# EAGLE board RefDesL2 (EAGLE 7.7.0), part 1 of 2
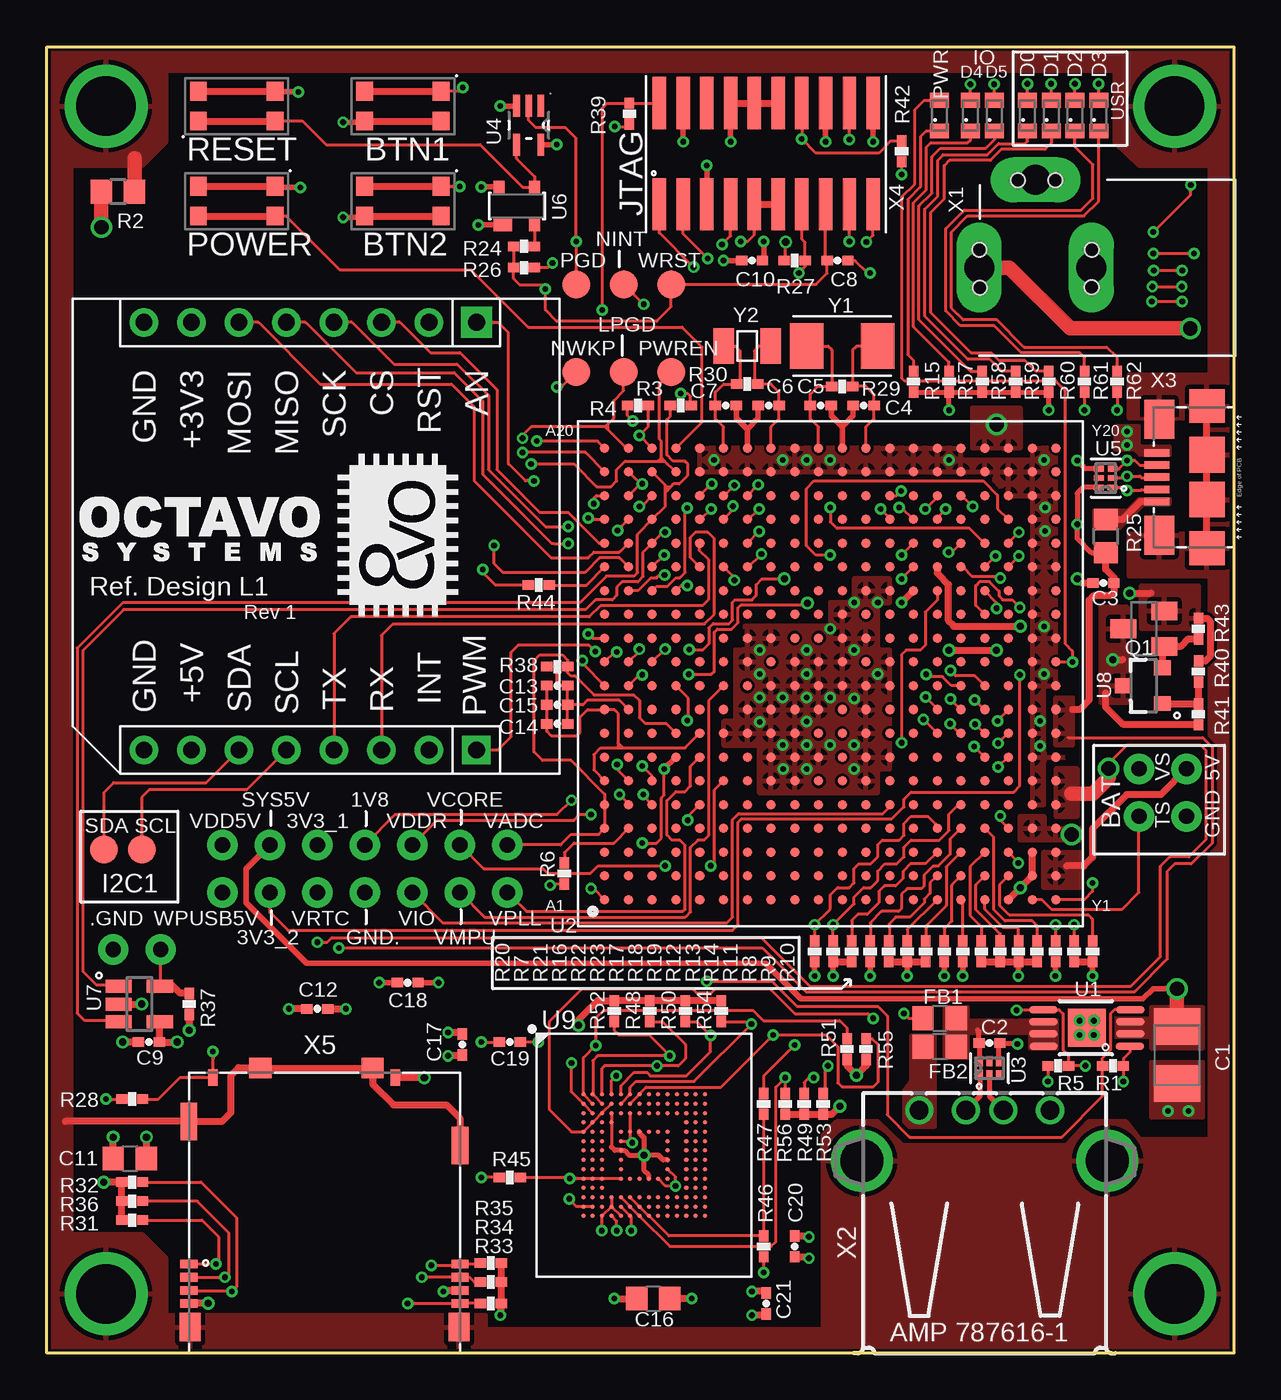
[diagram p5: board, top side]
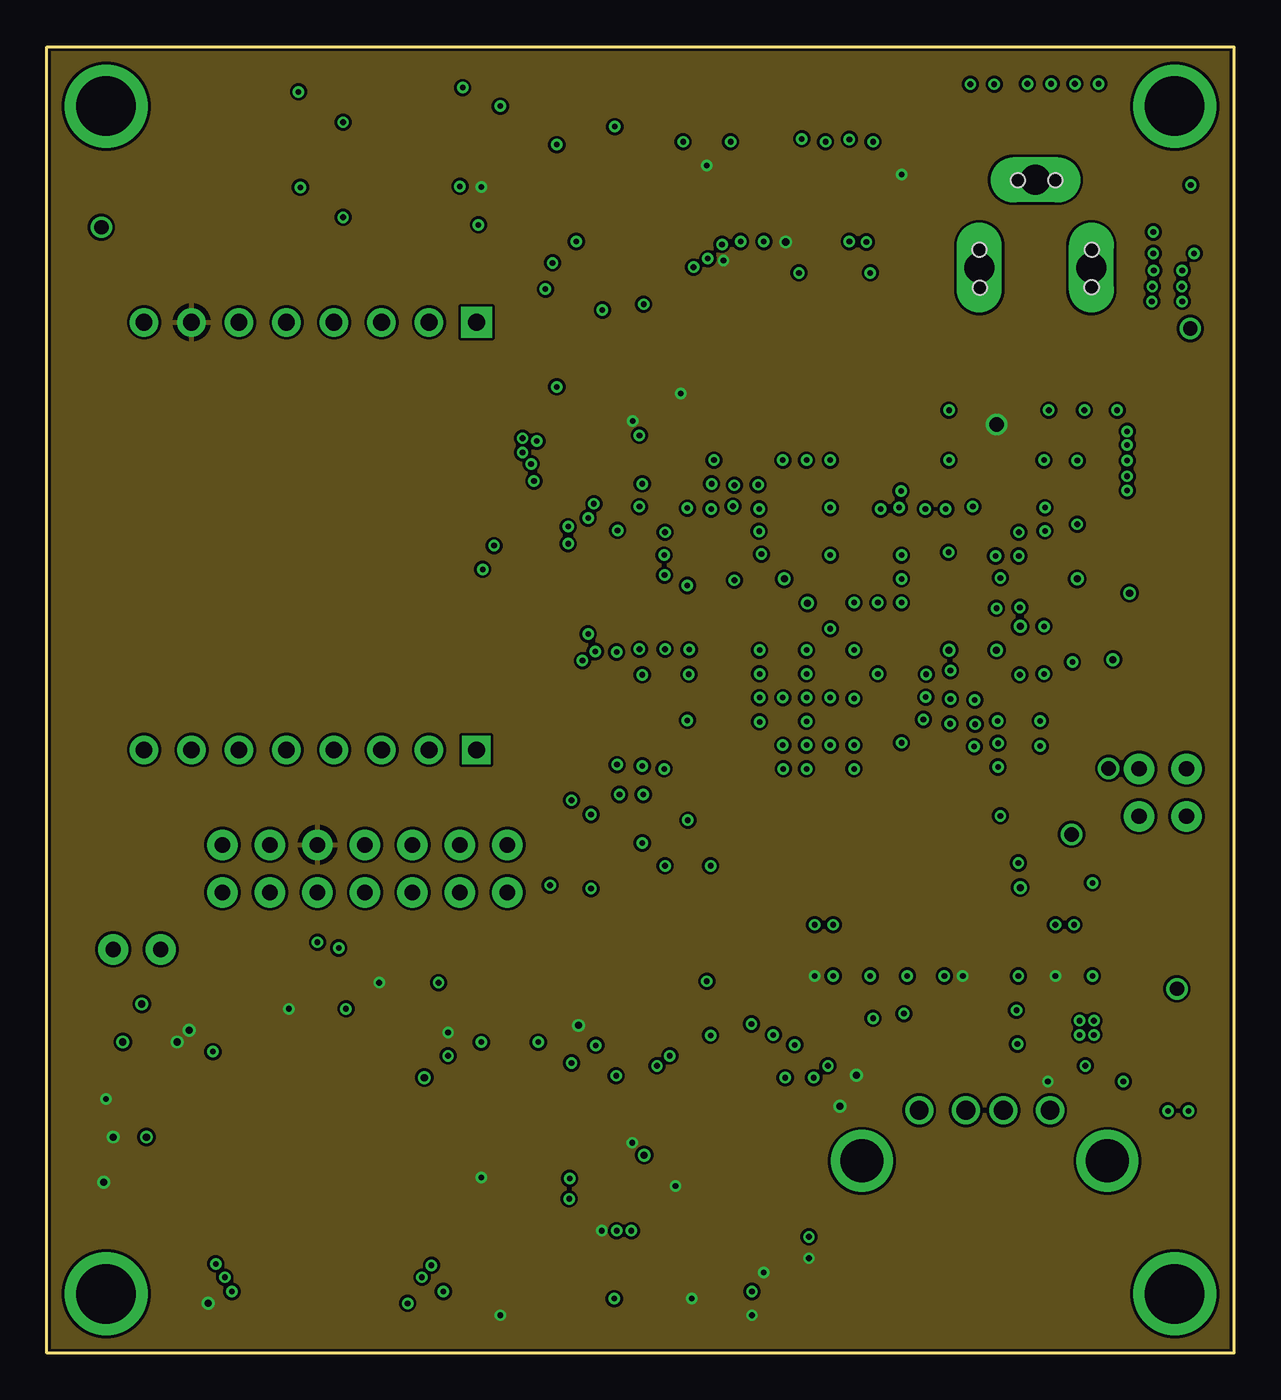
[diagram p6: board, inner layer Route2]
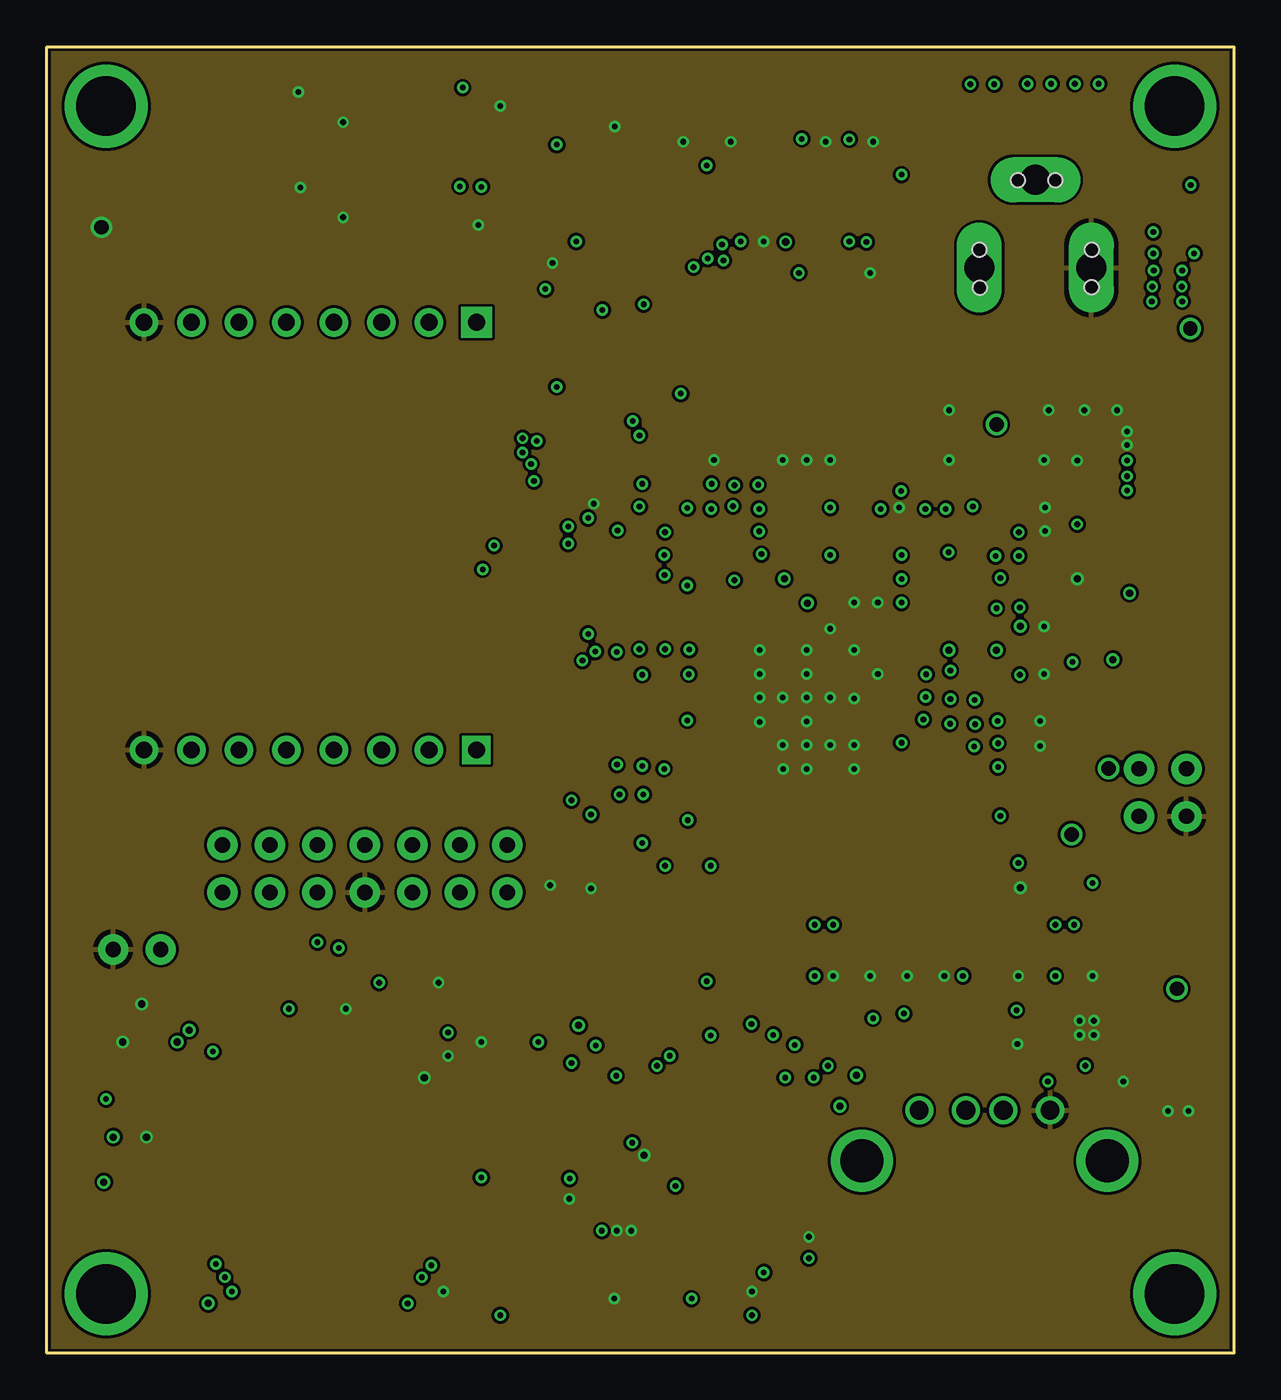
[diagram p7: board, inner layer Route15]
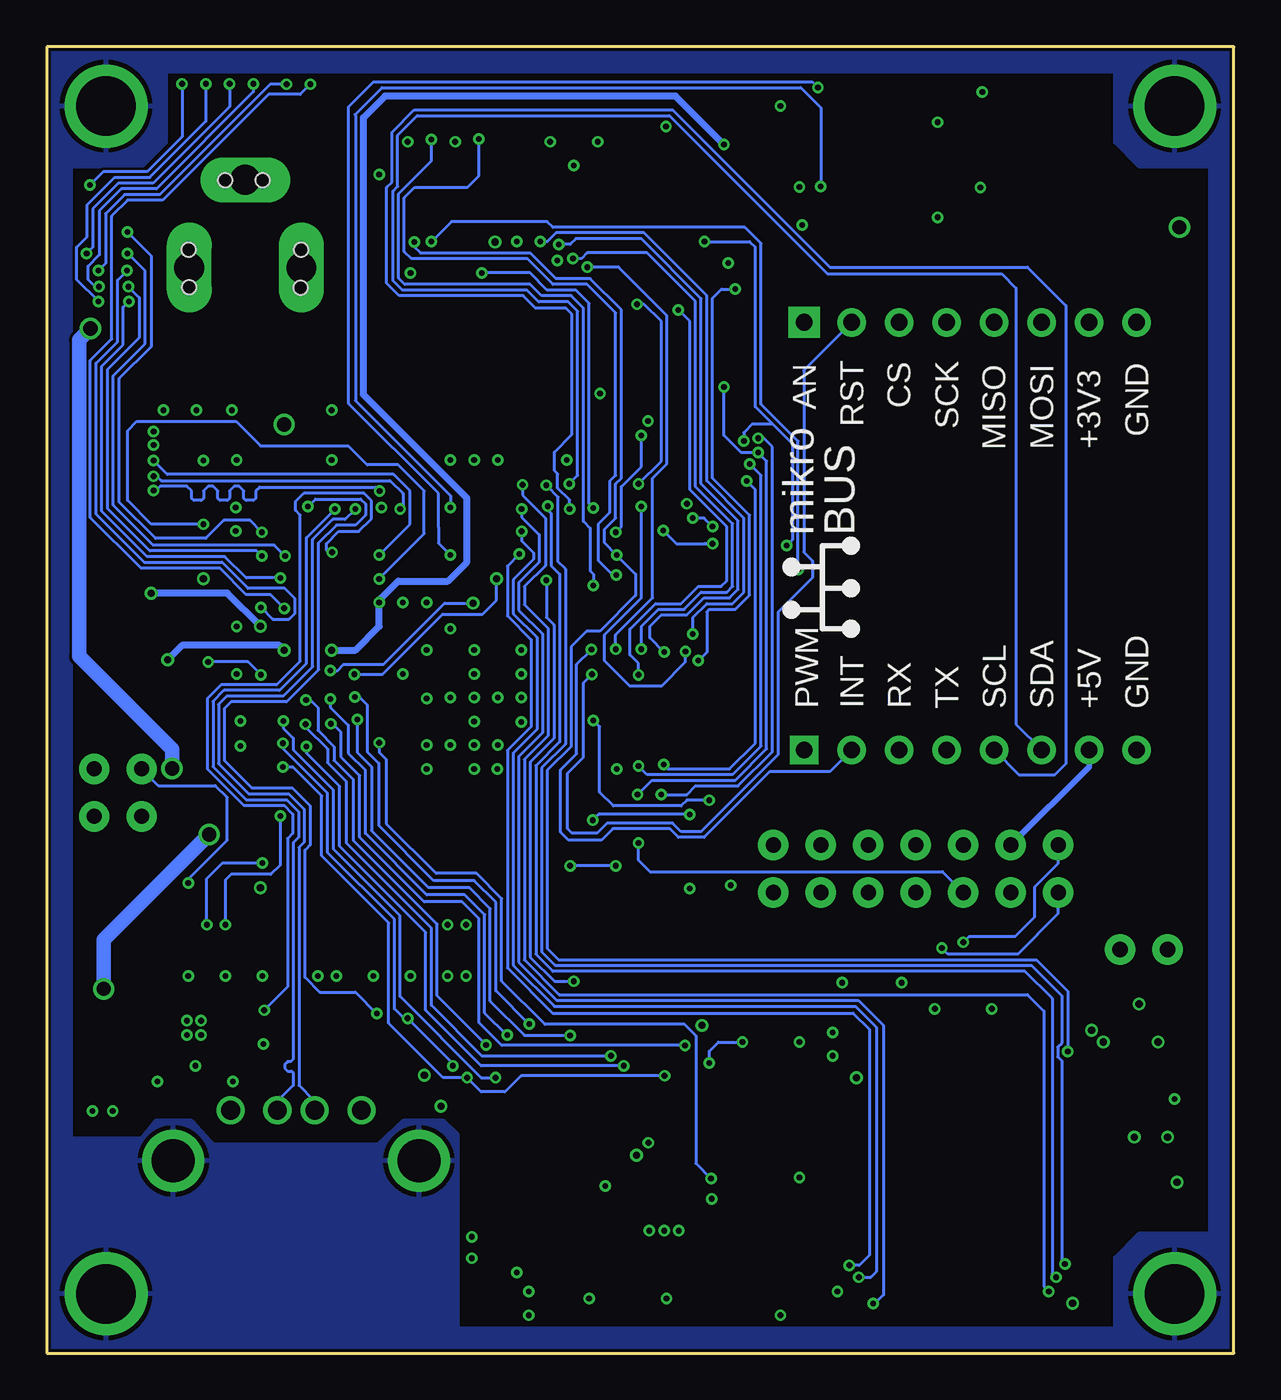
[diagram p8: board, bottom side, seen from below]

Size 63.5 x 69.85 mm. Coordinates in mm from the lower left corner, seen from the top.
Outline: 0,69.85 63.5,69.85 63.5,0 0,0 0,69.85
Copper layers (1+2*15+16): Top 0.07mm / dielectric 0.23mm / Route2 0.035mm / dielectric 0.93mm / Route15 0.035mm / dielectric 0.23mm / Bottom 0.07mm
Design rules "default *": minimum track width 6mil, minimum drill 12mil, track to track 6mil, track to pad 6mil, pad to pad 6mil, via to via 6mil, smd to smd 0mil, copper to edge 6mil, drill to drill 6mil, minimum pad ring 6mil, minimum via ring 6mil, stop-mask expansion 2mil, vias tented up to drill 25mil, thermal gap 10mil
Net classes: 0 default: width 0.127 mm, drill 0.254 mm

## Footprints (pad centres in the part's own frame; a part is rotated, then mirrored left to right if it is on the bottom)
TESTPAD/W_HOLE_1X1 = drill 0.813 pad 1.626: P$1 0,0
SW4SMD_63X161LS = smd 0.9 x 1: 1 2.05,0.8; 2 2.05,-0.8; 3 -2.05,0.8; 4 -2.05,-0.8
B/3528-21R = smd 1.95 x 2.5: + 1.525,0; - -1.525,0
C0402 = smd 0.61 x 0.508: 1 -0.559,0; 2 0.559,0
C0805 = smd 1.143 x 1.27: 1 -0.889,0; 2 0.889,0
EIA-STD = smd 0.787 x 1.016: 1 -0.826,0; 2 0.826,0
TP15R = smd 1.5 x 1.5: TP 0,0
MOUNTING_HOLE = drill 3.175 pad 4.445: P$1 0,0
SOT23-BEC = smd 1 x 1.4: B -0.95,-1.1; C 0,1.1; E 0.95,-1.1
R0402 = smd 0.61 x 0.508: 1 -0.559,0; 2 0.559,0
R0805 = smd 1.143 x 1.27: 1 -0.889,0; 2 0.889,0
S-PDSO-G08 = smd 1.524 x 0.406: 1 -2.311,0.975; 2 -2.324,0.325; 3 -2.324,-0.325; 4 -2.324,-0.975; 5 2.324,-0.975; 6 2.324,-0.325; 7 2.324,0.325; 8 2.311,0.975 | smd 2.032 x 2.032: TH 0,0
OSD335X-BGA-400 = smd 0.5 x 0.5: A1 -12.065,-12.065; A2 -12.065,-10.795; A3 -12.065,-9.525; A4 -12.065,-8.255; A5 -12.065,-6.985; A6 -12.065,-5.715; A7 -12.065,-4.445; A8 -12.065,-3.175; A9 -12.065,-1.905; A10 -12.065,-0.635; A11 -12.065,0.635; A12 -12.065,1.905; A13 -12.065,3.175; A14 -12.065,4.445; A15 -12.065,5.715; A16 -12.065,6.985; A17 -12.065,8.255; A18 -12.065,9.525; A19 -12.065,10.795; A20 -12.065,12.065; B1 -10.795,-12.065; B2 -10.795,-10.795; B3 -10.795,-9.525; B4 -10.795,-8.255; B5 -10.795,-6.985; B6 -10.795,-5.715; B7 -10.795,-4.445; B8 -10.795,-3.175; B9 -10.795,-1.905; B10 -10.795,-0.635; B11 -10.795,0.635; B12 -10.795,1.905; B13 -10.795,3.175; B14 -10.795,4.445; B15 -10.795,5.715; B16 -10.795,6.985; B17 -10.795,8.255; B18 -10.795,9.525; B19 -10.795,10.795; B20 -10.795,12.065; C1 -9.525,-12.065; C2 -9.525,-10.795; C3 -9.525,-9.525; C4 -9.525,-8.255; C5 -9.525,-6.985; C6 -9.525,-5.715; C7 -9.525,-4.445; C8 -9.525,-3.175; C9 -9.525,-1.905; C10 -9.525,-0.635; C11 -9.525,0.635; C12 -9.525,1.905; C13 -9.525,3.175; C14 -9.525,4.445; C15 -9.525,5.715; C16 -9.525,6.985; C17 -9.525,8.255; C18 -9.525,9.525; C19 -9.525,10.795; C20 -9.525,12.065; D1 -8.255,-12.065; D2 -8.255,-10.795; D3 -8.255,-9.525; D4 -8.255,-8.255; D5 -8.255,-6.985; D6 -8.255,-5.715; D7 -8.255,-4.445; D8 -8.255,-3.175; D9 -8.255,-1.905; D10 -8.255,-0.635; D11 -8.255,0.635; D12 -8.255,1.905; D13 -8.255,3.175; D14 -8.255,4.445; D15 -8.255,5.715; D16 -8.255,6.985; D17 -8.255,8.255; D18 -8.255,9.525; D19 -8.255,10.795; D20 -8.255,12.065; E1 -6.985,-12.065; E2 -6.985,-10.795; E3 -6.985,-9.525; E4 -6.985,-8.255; E5 -6.985,-6.985; E6 -6.985,-5.715; E7 -6.985,-4.445; E8 -6.985,-3.175; E9 -6.985,-1.905; E10 -6.985,-0.635; E11 -6.985,0.635; E12 -6.985,1.905; E13 -6.985,3.175; E14 -6.985,4.445; E15 -6.985,5.715; E16 -6.985,6.985; E17 -6.985,8.255; E18 -6.985,9.525; E19 -6.985,10.795; E20 -6.985,12.065; F1 -5.715,-12.065; F2 -5.715,-10.795; F3 -5.715,-9.525; F4 -5.715,-8.255; F5 -5.715,-6.985; F6 -5.715,-5.715; F7 -5.715,-4.445; F8 -5.715,-3.175; F9 -5.715,-1.905; F10 -5.715,-0.635; F11 -5.715,0.635; F12 -5.715,1.905; F13 -5.715,3.175; F14 -5.715,4.445; F15 -5.715,5.715; F16 -5.715,6.985; F17 -5.715,8.255; F18 -5.715,9.525; F19 -5.715,10.795; F20 -5.715,12.065; G1 -4.445,-12.065; G2 -4.445,-10.795; G3 -4.445,-9.525; G4 -4.445,-8.255; G5 -4.445,-6.985; G6 -4.445,-5.715; G7 -4.445,-4.445; G8 -4.445,-3.175; G9 -4.445,-1.905; G10 -4.445,-0.635; G11 -4.445,0.635; G12 -4.445,1.905; G13 -4.445,3.175; G14 -4.445,4.445; G15 -4.445,5.715; G16 -4.445,6.985; G17 -4.445,8.255; G18 -4.445,9.525; G19 -4.445,10.795; G20 -4.445,12.065; H1 -3.175,-12.065; H2 -3.175,-10.795; H3 -3.175,-9.525; H4 -3.175,-8.255; H5 -3.175,-6.985; H6 -3.175,-5.715; H7 -3.175,-4.445; H8 -3.175,-3.175; H9 -3.175,-1.905; H10 -3.175,-0.635; H11 -3.175,0.635; H12 -3.175,1.905; H13 -3.175,3.175; H14 -3.175,4.445; H15 -3.175,5.715; H16 -3.175,6.985; H17 -3.175,8.255; H18 -3.175,9.525; H19 -3.175,10.795; H20 -3.175,12.065; J1 -1.905,-12.065; J2 -1.905,-10.795; J3 -1.905,-9.525; J4 -1.905,-8.255; J5 -1.905,-6.985; J6 -1.905,-5.715; J7 -1.905,-4.445; J8 -1.905,-3.175; J9 -1.905,-1.905; J10 -1.905,-0.635; J11 -1.905,0.635; J12 -1.905,1.905; J13 -1.905,3.175; J14 -1.905,4.445; J15 -1.905,5.715; J16 -1.905,6.985; J17 -1.905,8.255; J18 -1.905,9.525; J19 -1.905,10.795; J20 -1.905,12.065; K1 -0.635,-12.065; K2 -0.635,-10.795; K3 -0.635,-9.525; K4 -0.635,-8.255; K5 -0.635,-6.985; K6 -0.635,-5.715; K7 -0.635,-4.445; K8 -0.635,-3.175; K9 -0.635,-1.905; K10 -0.635,-0.635; K11 -0.635,0.635; K12 -0.635,1.905; K13 -0.635,3.175; K14 -0.635,4.445; K15 -0.635,5.715; K16 -0.635,6.985; K17 -0.635,8.255; K18 -0.635,9.525; K19 -0.635,10.795; K20 -0.635,12.065; L1 0.635,-12.065; L2 0.635,-10.795; L3 0.635,-9.525; L4 0.635,-8.255; L5 0.635,-6.985; L6 0.635,-5.715; L7 0.635,-4.445; L8 0.635,-3.175; L9 0.635,-1.905; L10 0.635,-0.635; L11 0.635,0.635; L12 0.635,1.905; L13 0.635,3.175; L14 0.635,4.445; L15 0.635,5.715; L16 0.635,6.985; L17 0.635,8.255; L18 0.635,9.525; L19 0.635,10.795; L20 0.635,12.065; M1 1.905,-12.065; M2 1.905,-10.795; M3 1.905,-9.525; M4 1.905,-8.255; M5 1.905,-6.985; M6 1.905,-5.715; M7 1.905,-4.445; M8 1.905,-3.175; M9 1.905,-1.905; M10 1.905,-0.635; M11 1.905,0.635; M12 1.905,1.905; M13 1.905,3.175; M14 1.905,4.445; M15 1.905,5.715; M16 1.905,6.985; M17 1.905,8.255; M18 1.905,9.525; M19 1.905,10.795; M20 1.905,12.065; N1 3.175,-12.065; N2 3.175,-10.795; N3 3.175,-9.525; N4 3.175,-8.255; N5 3.175,-6.985; N6 3.175,-5.715; N7 3.175,-4.445; N8 3.175,-3.175; N9 3.175,-1.905; N10 3.175,-0.635; N11 3.175,0.635; N12 3.175,1.905; N13 3.175,3.175; N14 3.175,4.445; N15 3.175,5.715; N16 3.175,6.985; N17 3.175,8.255; N18 3.175,9.525; N19 3.175,10.795; N20 3.175,12.065; P1 4.445,-12.065; P2 4.445,-10.795; P3 4.445,-9.525; P4 4.445,-8.255; P5 4.445,-6.985; P6 4.445,-5.715; P7 4.445,-4.445; P8 4.445,-3.175; P9 4.445,-1.905; P10 4.445,-0.635; P11 4.445,0.635; P12 4.445,1.905; P13 4.445,3.175; P14 4.445,4.445; P15 4.445,5.715; P16 4.445,6.985; P17 4.445,8.255; P18 4.445,9.525; P19 4.445,10.795; P20 4.445,12.065; R1 5.715,-12.065; R2 5.715,-10.795; R3 5.715,-9.525; R4 5.715,-8.255; R5 5.715,-6.985; R6 5.715,-5.715; R7 5.715,-4.445; R8 5.715,-3.175; R9 5.715,-1.905; R10 5.715,-0.635; R11 5.715,0.635; R12 5.715,1.905; R13 5.715,3.175; R14 5.715,4.445; R15 5.715,5.715; R16 5.715,6.985; R17 5.715,8.255; R18 5.715,9.525; R19 5.715,10.795; R20 5.715,12.065; T1 6.985,-12.065; T2 6.985,-10.795; T3 6.985,-9.525; T4 6.985,-8.255; T5 6.985,-6.985; T6 6.985,-5.715; T7 6.985,-4.445; T8 6.985,-3.175; T9 6.985,-1.905; T10 6.985,-0.635; T11 6.985,0.635; T12 6.985,1.905; T13 6.985,3.175; T14 6.985,4.445; T15 6.985,5.715; T16 6.985,6.985; T17 6.985,8.255; T18 6.985,9.525; T19 6.985,10.795; T20 6.985,12.065; U1 8.255,-12.065; U2 8.255,-10.795; U3 8.255,-9.525; U4 8.255,-8.255; U5 8.255,-6.985; U6 8.255,-5.715; U7 8.255,-4.445; U8 8.255,-3.175; U9 8.255,-1.905; U10 8.255,-0.635; U11 8.255,0.635; U12 8.255,1.905; U13 8.255,3.175; U14 8.255,4.445; U15 8.255,5.715; U16 8.255,6.985; U17 8.255,8.255; U18 8.255,9.525; U19 8.255,10.795; U20 8.255,12.065; V1 9.525,-12.065; V2 9.525,-10.795; V3 9.525,-9.525; V4 9.525,-8.255; V5 9.525,-6.985; V6 9.525,-5.715; V7 9.525,-4.445; V8 9.525,-3.175; V9 9.525,-1.905; V10 9.525,-0.635; V11 9.525,0.635; V12 9.525,1.905; V13 9.525,3.175; V14 9.525,4.445; V15 9.525,5.715; V16 9.525,6.985; V17 9.525,8.255; V18 9.525,9.525; V19 9.525,10.795; V20 9.525,12.065; W1 10.795,-12.065; W2 10.795,-10.795; W3 10.795,-9.525; W4 10.795,-8.255; W5 10.795,-6.985; W6 10.795,-5.715; W7 10.795,-4.445; W8 10.795,-3.175; W9 10.795,-1.905; W10 10.795,-0.635; W11 10.795,0.635; W12 10.795,1.905; W13 10.795,3.175; W14 10.795,4.445; W15 10.795,5.715; W16 10.795,6.985; W17 10.795,8.255; W18 10.795,9.525; W19 10.795,10.795; W20 10.795,12.065; Y1 12.065,-12.065; Y2 12.065,-10.795; Y3 12.065,-9.525; Y4 12.065,-8.255; Y5 12.065,-6.985; Y6 12.065,-5.715; Y7 12.065,-4.445; Y8 12.065,-3.175; Y9 12.065,-1.905; Y10 12.065,-0.635; Y11 12.065,0.635; Y12 12.065,1.905; Y13 12.065,3.175; Y14 12.065,4.445; Y15 12.065,5.715; Y16 12.065,6.985; Y17 12.065,8.255; Y18 12.065,9.525; Y19 12.065,10.795; Y20 12.065,12.065
DRY6 = smd 0.55 x 0.3: 1 -0.355,0.5 | smd 0.52 x 0.3: 2 -0.37,0; 3 -0.37,-0.5; 4 0.37,-0.5; 5 0.37,0; 6 0.37,0.5
DCK5 = smd 1.168 x 0.356: 1 -1.041,0.65; 2 -1.041,0; 3 -1.041,-0.65; 4 1.041,-0.65; 5 1.041,0.65
SOT143-R = smd 1 x 0.7: 1 -0.75,-1 | smd 0.6 x 0.7: 2 0.95,-1; 3 0.95,1; 4 -0.95,1
SOT23-5 = smd 0.7 x 1.4: 1 0.95,1.1; 2 0,1.1; 3 -0.95,1.1; 4 -0.95,-1.1; 5 0.95,-1.1
SOT23-3 = smd 0.8 x 0.9: 1 -0.95,-1; 2 0.95,-1; 3 0,1.1
MICRON_EMMC_153 = smd 0.245 x 0.245: A1 -3.25,3.25; A2 -2.75,3.25; A3 -2.25,3.25; A4 -1.75,3.25; A5 -1.25,3.25; A6 -0.75,3.25; A7 -0.25,3.25; A8 0.25,3.25; A9 0.75,3.25; A10 1.25,3.25; A11 1.75,3.25; A12 2.25,3.25; A13 2.75,3.25; A14 3.25,3.25; B1 -3.25,2.75; B2 -2.75,2.75; B3 -2.25,2.75; B4 -1.75,2.75; B5 -1.25,2.75; B6 -0.75,2.75; B7 -0.25,2.75; B8 0.25,2.75; B9 0.75,2.75; B10 1.25,2.75; B11 1.75,2.75; B12 2.25,2.75; B13 2.75,2.75; B14 3.25,2.75; C1 -3.25,2.25; C2 -2.75,2.25; C3 -2.25,2.25; C4 -1.75,2.25; C5 -1.25,2.25; C6 -0.75,2.25; C7 -0.25,2.25; C8 0.25,2.25; C9 0.75,2.25; C10 1.25,2.25; C11 1.75,2.25; C12 2.25,2.25; C13 2.75,2.25; C14 3.25,2.25; D1 -3.25,1.75; D2 -2.75,1.75; D3 -2.25,1.75; D4 -1.75,1.75; D12 2.25,1.75; D13 2.75,1.75; D14 3.25,1.75; E1 -3.25,1.25; E2 -2.75,1.25; E3 -2.25,1.25; E5 -1.25,1.25; E6 -0.75,1.25; E7 -0.25,1.25; E8 0.25,1.25; E9 0.75,1.25; E10 1.25,1.25; E12 2.25,1.25; E13 2.75,1.25; E14 3.25,1.25; F1 -3.25,0.75; F2 -2.75,0.75; F3 -2.25,0.75; F5 -1.25,0.75; F10 1.25,0.75; F12 2.25,0.75; F13 2.75,0.75; F14 3.25,0.75; G1 -3.25,0.25; G2 -2.75,0.25; G3 -2.25,0.25; G5 -1.25,0.25; G10 1.25,0.25; G12 2.25,0.25; G13 2.75,0.25; G14 3.25,0.25; H1 -3.25,-0.25; H2 -2.75,-0.25; H3 -2.25,-0.25; H5 -1.25,-0.25; H10 1.25,-0.25; H12 2.25,-0.25; H13 2.75,-0.25; H14 3.25,-0.25; J1 -3.25,-0.75; J2 -2.75,-0.75; J3 -2.25,-0.75; J5 -1.25,-0.75; J10 1.25,-0.75; J12 2.25,-0.75; J13 2.75,-0.75; J14 3.25,-0.75; K1 -3.25,-1.25; K2 -2.75,-1.25; K3 -2.25,-1.25; K5 -1.25,-1.25; K6 -0.75,-1.25; K7 -0.25,-1.25; K8 0.25,-1.25; K9 0.75,-1.25; K10 1.25,-1.25; K12 2.25,-1.25; K13 2.75,-1.25; K14 3.25,-1.25; L1 -3.25,-1.75; L2 -2.75,-1.75; L3 -2.25,-1.75; L12 2.25,-1.75; L13 2.75,-1.75; L14 3.25,-1.75; M1 -3.25,-2.25; M2 -2.75,-2.25; M3 -2.25,-2.25; M4 -1.75,-2.25; M5 -1.25,-2.25; M6 -0.75,-2.25; M7 -0.25,-2.25; M8 0.25,-2.25; M9 0.75,-2.25; M10 1.25,-2.25; M11 1.75,-2.25; M12 2.25,-2.25; M13 2.75,-2.25; M14 3.25,-2.25; N1 -3.25,-2.75; N2 -2.75,-2.75; N3 -2.25,-2.75; N4 -1.75,-2.75; N5 -1.25,-2.75; N6 -0.75,-2.75; N7 -0.25,-2.75; N8 0.25,-2.75; N9 0.75,-2.75; N10 1.25,-2.75; N11 1.75,-2.75; N12 2.25,-2.75; N13 2.75,-2.75; N14 3.25,-2.75; P1 -3.25,-3.25; P2 -2.75,-3.25; P3 -2.25,-3.25; P4 -1.75,-3.25; P5 -1.25,-3.25; P6 -0.75,-3.25; P7 -0.25,-3.25; P8 0.25,-3.25; P9 0.75,-3.25; P10 1.25,-3.25; P11 1.75,-3.25; P12 2.25,-3.25; P13 2.75,-3.25; P14 3.25,-3.25
PJ-102B_POWER_CON = drill 1.6 long: IN -6,0; OUT 0,0; OUT_CON -3,4.7 | hole 0.762: 0,-1.041; 0.025,0.965; -5.994,0.965; -5.969,-1.067; -1.93,4.674; -3.937,4.674
USB_HOST_HORIZONTAL_W/CHASSIS_GND = drill 1: 1 -3.5,12.99; 2 -1,12.99; 3 1,12.99; 4 3.5,12.99 | drill 2.3: 5 -6.57,10.28; 6 6.57,10.28
10118192-0001LF(MICRO-USB-B-AMPHENOL-FCI) = smd 1.8 x 1.9: CGND1 -3.8,0; CGND4 3.8,0 | smd 1.9 x 1.9: CGND2 -1.2,0; CGND3 1.2,0 | smd 2.1 x 1.6: CGND5 3.1,2.55; CGND6 -3.1,2.55 | smd 0.4 x 1.35: D+ 0,2.675; D- -0.65,2.675; GND 1.3,2.675; ID 0.65,2.675; VBUS -1.3,2.675
CTI-JTAG = smd 2.794 x 0.711: 1 -2.705,5.715; 2 2.705,5.715; 3 -2.705,4.445; 4 2.705,4.445; 5 -2.705,3.175; 6 2.705,3.175; 7 -2.705,1.905; 8 2.705,1.905; 9 -2.705,0.635; 10 2.705,0.635; 11 -2.705,-0.635; 12 2.705,-0.635; 13 -2.705,-1.905; 14 2.705,-1.905; 15 -2.705,-3.175; 16 2.705,-3.175; 17 -2.705,-4.445; 18 2.705,-4.445; 19 -2.705,-5.715; 20 2.705,-5.715
SCHA5B0200 = smd 0.915 x 0.458: 1 -7.257,3.365; 2 -7.257,2.665; 3 -7.257,1.965; 4 -7.257,1.265; 5 7.257,1.265; 6 7.257,1.965; 7 7.257,2.665; 8 7.257,3.365 | smd 0.51 x 0.887: CD -5.975,13.354; GND 3.775,13.354 | smd 0.891 x 2.007: CGND1 -7.25,11; CGND4 7.25,9.7 | smd 1.117 x 1.525: CGND2 -7.196,0; CGND3 7.196,0 | smd 1.192 x 1.092: CGND5 2.575,13.853; CGND6 -3.425,13.853
MIKROE_BUS_MINI = drill 0.889 pad 1.676 square: 1 1.27,21.59 | drill 0.889 pad 1.524: 2 1.27,19.05; 3 1.27,16.51; 4 1.27,13.97; 5 1.27,11.43; 6 1.27,8.89; 7 1.27,6.35; 8 1.27,3.81; 9 24.13,3.81; 10 24.13,6.35; 11 24.13,8.89; 12 24.13,11.43; 13 24.13,13.97; 14 24.13,16.51; 15 24.13,19.05 | drill 0.889 pad 1.524 square: 16 24.13,21.59
CRYSTAL-TXC-7A = smd 1.788 x 2.413: P$1 1.9,0; P$2 -1.9,0
CRYSTAL_3.2X1.5 = smd 1.1 x 1.9: P$1 -1.25,0; P$2 1.25,0

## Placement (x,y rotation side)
1V8  TESTPAD/W_HOLE_1X1  [TESTPAD/W_HOLE_1X1]  17.02,27.18 0 top
3V3_1  TESTPAD/W_HOLE_1X1  [TESTPAD/W_HOLE_1X1]  14.48,27.18 0 top
3V3_2  TESTPAD/W_HOLE_1X1  [TESTPAD/W_HOLE_1X1]  11.94,24.64 0 top
.GND  TESTPAD/W_HOLE_1X1  [TESTPAD/W_HOLE_1X1]  3.56,21.59 0 top
BAT5V  TESTPAD/W_HOLE_1X1  [TESTPAD/W_HOLE_1X1]  60.96,31.24 0 top
BAT_T  TESTPAD/W_HOLE_1X1  [TESTPAD/W_HOLE_1X1]  58.42,28.7 0 top
BAT_V  TESTPAD/W_HOLE_1X1  [TESTPAD/W_HOLE_1X1]  58.42,31.24 0 top
BTN1  KMR231GLFS  [SW4SMD_63X161LS]  19.05,66.67 0 top
BTN2  KMR231GLFS  [SW4SMD_63X161LS]  19.05,61.59 0 top
C1  220uF, 6.3V  [B/3528-21R]  60.45,15.94 90 top
C2  0.1uF, 6.3V  [C0402]  50.42,16.59 0 top
C3  0.1uF, 6.3V  [C0402]  56.52,41.17 180 top
C4  18pF, 50V  [C0402]  43.69,50.67 180 top
C5  18pF, 50V  [C0402]  41.4,50.67 0 top
C6  18pF, 50V  [C0402]  38.61,50.67 180 top
C7  18pF, 50V  [C0402]  36.32,50.67 0 top
C8  0.1uF, 6.3V  [C0402]  42.29,58.42 0 top
C9  0.1uF, 6.3V  [C0402]  5.46,16.64 0 top
C10  0.1uF, 6.3V  [C0402]  37.72,58.42 0 top
C11  10uF, 10V  [C0805]  4.45,10.41 0 top
C12  0.1uF, 6.3V  [C0402]  14.48,18.41 0 top
C13  0.1uF, 6.3V  [C0402]  27.3,35.69 180 top
C14  0.1uF, 6.3V  [C0402]  27.3,33.66 180 top
C15  .001uF, 50V  [C0402]  27.3,34.67 180 top
C16  10uF, 10V  [C0805]  32.44,2.92 0 top
C17  0.1uF, 6.3V  [C0402]  22.23,16.51 90 top
C18  0.1uF, 6.3V  [C0402]  19.3,19.81 180 top
C19  2.2uF  [C0402]  24.77,16.64 180 top
C20  0.1uF, 6.3V  [C0402]  40.01,5.71 270 top
C21  0.1uF, 6.3V  [C0402]  38.48,2.67 270 top
D0  LTST-C191TBKT  [EIA-STD]  52.45,66.17 270 top
D1  LTST-C191TBKT  [EIA-STD]  53.72,66.17 270 top
D2  LTST-C191TBKT  [EIA-STD]  54.99,66.17 270 top
D3  LTST-C191TBKT  [EIA-STD]  56.26,66.17 270 top
D4  LTST-C191TBKT  [EIA-STD]  49.4,66.17 270 top
D5  LTST-C191TBKT  [EIA-STD]  50.67,66.17 270 top
FB1  0.1Ohm, 0805  [C0805]  47.75,17.91 0 top
FB2  150Ohm, 800mA  [C0805]  47.75,16.38 180 top
GND  TESTPAD/W_HOLE_1X1  [TESTPAD/W_HOLE_1X1]  60.96,28.7 0 top
GND.  TESTPAD/W_HOLE_1X1  [TESTPAD/W_HOLE_1X1]  17.02,24.64 0 top
I2C0_SDA  TPTP15R  [TP15R]  3.05,26.92 0 top
I2C1_SCL  TPTP15R  [TP15R]  5.08,26.92 0 top
LPGD  TPTP15R  [TP15R]  30.86,52.45 0 top
MGT1  MOUNTING_HOLE  [MOUNTING_HOLE]  60.33,3.17 0 top
MGT2  MOUNTING_HOLE  [MOUNTING_HOLE]  60.33,66.67 0 top
MGT3  MOUNTING_HOLE  [MOUNTING_HOLE]  3.17,66.67 0 top
MGT4  MOUNTING_HOLE  [MOUNTING_HOLE]  3.17,3.17 0 top
NINT  TPTP15R  [TP15R]  30.86,57.15 0 top
NWKP  TPTP15R  [TP15R]  28.32,52.45 0 top
PGD  TPTP15R  [TP15R]  28.32,57.15 0 top
POWER  KMR231GLFS  [SW4SMD_63X161LS]  10.16,61.59 0 top
PWR  LTST-C191TBKT  [EIA-STD]  47.75,66.17 270 top
PWREN  TPTP15R  [TP15R]  33.4,52.45 0 top
Q1  MMBT2907  [SOT23-BEC]  58.67,38.73 90 top
R1  10K  [R0402]  57.02,15.37 180 top
R2  0.1, 5%  [R0805]  3.81,62.1 180 top
R3  1.5K, 1%  [R0402]  33.91,50.67 0 top
R4  1.5K, 1%  [R0402]  31.62,50.67 180 top
R5  10K  [R0402]  54.1,15.37 180 top
R6  10K  [R0402]  27.69,25.65 270 top
R7  100K, 1%  [R0402]  42.06,21.49 90 top
R8  100K, 1%  [R0402]  53.95,21.49 270 top
R9  100K, 1%  [R0402]  54.94,21.49 90 top
R10  100K, 1%  [R0402]  55.93,21.49 90 top
R11  100K, 1%  [R0402]  52.96,21.49 90 top
R12  100K, 1%  [R0402]  49.99,21.49 90 top
R13  100K, 1%  [R0402]  50.98,21.49 90 top
R14  100K, 1%  [R0402]  51.97,21.49 90 top
R15  1.5K, 1%  [R0402]  46.35,51.94 270 top
R16  100K, 1%  [R0402]  44.04,21.49 90 top
R17  100K, 1%  [R0402]  47.02,21.49 90 top
R18  100K, 1%  [R0402]  48.01,21.49 90 top
R19  100K, 1%  [R0402]  49,21.49 270 top
R20  100K, 1%  [R0402]  41.07,21.49 270 top
R21  100K, 1%  [R0402]  43.05,21.49 90 top
R22  100K, 1%  [R0402]  45.03,21.49 90 top
R23  100K, 1%  [R0402]  46.02,21.49 90 top
R24  1K  [R0402]  25.53,59.18 0 top
R25  0, 1%  [R0805]  56.64,43.69 90 top
R26  100K, DNI  [R0402]  25.53,58.04 180 top
R27  4.75K, 1%  [R0402]  40.01,58.42 180 top
R28  10K  [R0402]  4.57,13.59 180 top
R29  1M, 1%  [R0402]  42.55,51.69 0 top
R30  1M, DNI  [R0402]  37.47,51.82 0 top
R31  10K  [R0402]  4.57,7.11 180 top
R32  10K  [R0402]  4.57,9.14 180 top
R33  10K  [R0402]  23.75,2.67 0 top
R34  10K  [R0402]  23.75,3.81 0 top
R35  10K  [R0402]  23.75,4.83 0 top
R36  10K  [R0402]  4.57,8.13 180 top
R37  10K  [R0402]  7.62,18.67 90 top
R38  0, 1%  [R0402]  27.3,36.7 0 top
R39  4.75K, 1%  [R0402]  31.17,66.27 90 top
R40  10K  [R0402]  61.59,36.45 90 top
R41  40.2K, 1%  [R0402]  61.59,34.16 90 top
R42  4.75K, 1%  [R0402]  45.72,64.26 270 top
R43  499  [R0402]  61.59,38.73 90 top
R44  33, 5%  [R0402]  26.31,41.07 180 top
R45  10K  [R0402]  24.77,9.4 180 top
R46  10K  [R0402]  38.35,5.71 270 top
R47  10K  [R0402]  39.5,13.34 270 top
R48  10K  [R0402]  32.26,18.29 90 top
R49  10K  [R0402]  40.51,13.34 270 top
R50  10K  [R0402]  34.16,18.29 90 top
R51  10K  [R0402]  42.8,16.26 270 top
R52  10K  [R0402]  30.35,18.29 90 top
R53  10K  [R0402]  41.53,13.34 270 top
R54  10K  [R0402]  36.07,18.29 90 top
R55  10K  [R0402]  43.81,16.26 270 top
R56  33, 5%  [R0402]  38.35,13.34 270 top
R57  1.5K  [R0402]  48.26,51.94 270 top
R58  1.5K  [R0402]  50.04,51.94 270 top
R59  1.5K  [R0402]  51.82,51.94 90 top
R60  1.5K  [R0402]  53.59,51.94 90 top
R61  1.5K  [R0402]  55.5,51.94 90 top
R62  1.5K  [R0402]  57.25,51.94 90 top
RESET  KMR231GLFS  [SW4SMD_63X161LS]  10.16,66.67 180 top
SYS5V  TESTPAD/W_HOLE_1X1  [TESTPAD/W_HOLE_1X1]  11.94,27.18 0 top
U1  TPS2051  [S-PDSO-G08]  55.63,17.4 180 top
U2  [OSD335X-BGA-400]  41.91,36.32 0 top
U3  TPD4S012_DRY_6  [DRY6]  50.42,15.24 90 top
U4  SN74LVC1G07_DCK_5  [DCK5]  25.78,65.66 270 top
U5  TPD4S012_DRY_6  [DRY6]  56.64,46.79 180 top
U6  APX811SOT  [SOT143-R]  25.15,61.34 0 top
U7  24LC32A  [SOT23-5]  4.95,18.67 90 top
U8  TLVH431  [SOT23-3]  58.67,35.69 90 top
U9  EMMC  [MICRON_EMMC_153]  31.95,10.59 0 top
U$1  [OCTAVO-LOGO]  1.65,39.24 0 top
USB5V  TESTPAD/W_HOLE_1X1  [TESTPAD/W_HOLE_1X1]  9.4,24.64 0 top
VADC  TESTPAD/W_HOLE_1X1  [TESTPAD/W_HOLE_1X1]  24.64,27.18 0 top
VCORE  TESTPAD/W_HOLE_1X1  [TESTPAD/W_HOLE_1X1]  22.1,27.18 0 top
VDD5V  TESTPAD/W_HOLE_1X1  [TESTPAD/W_HOLE_1X1]  9.4,27.18 0 top
VDDR  TESTPAD/W_HOLE_1X1  [TESTPAD/W_HOLE_1X1]  19.56,27.18 0 top
VIO  TESTPAD/W_HOLE_1X1  [TESTPAD/W_HOLE_1X1]  19.56,24.64 0 top
VMPU  TESTPAD/W_HOLE_1X1  [TESTPAD/W_HOLE_1X1]  22.1,24.64 0 top
VPLL  TESTPAD/W_HOLE_1X1  [TESTPAD/W_HOLE_1X1]  24.64,24.64 0 top
VRTC  TESTPAD/W_HOLE_1X1  [TESTPAD/W_HOLE_1X1]  14.48,24.64 0 top
WP  TESTPAD/W_HOLE_1X1  [TESTPAD/W_HOLE_1X1]  6.1,21.59 0 top
WRST  TPTP15R  [TP15R]  33.4,57.15 0 top
X1  PJ-102BH-PWR_CONN  [PJ-102B_POWER_CON]  55.88,58.04 0 top
X2  AMP 787616-1  [USB_HOST_HORIZONTAL_W/CHASSIS_GND]  50.16,0 0 top
X3  10118192-0001LF  [10118192-0001LF(MICRO-USB-B-AMPHENOL-FCI)]  62.05,46.84 90 top
X4  JTAG  [CTI-JTAG]  38.48,64.14 90 top
X5  SCHA5B0200(ALPS_USD)  [SCHA5B0200]  14.86,1.4 0 top
X6  MIKROE_CLICKMINI  [MIKROE_BUS_MINI]  1.4,56.39 270 top
Y1  7A-24.000MAAJ-T  [CRYSTAL-TXC-7A]  42.55,53.85 180 top
Y2  ABS07-32.768KHZ-T  [CRYSTAL_3.2X1.5]  37.47,53.85 0 top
